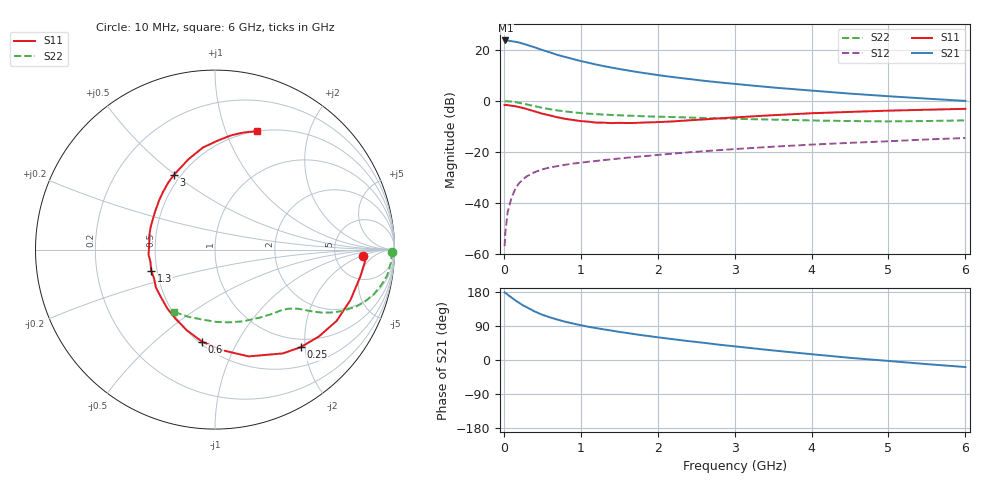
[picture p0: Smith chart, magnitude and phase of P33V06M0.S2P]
! SIEMENS Small Signal Semiconductors
! BFP181
! Si NPN RF Bipolar Junction Transistor in SOT143
! VCE = 3 V  IC = 6 mA
! Common Emitter S-Parameters:  March  1996
# GHz  S  MA  R  50
!  f  S11  S21  S12  S22
! GHz  MAG  ANG  MAG  ANG  MAG  ANG  MAG  ANG
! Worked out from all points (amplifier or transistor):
!   36 points, 10 MHz to 6 GHz, reference 50 ohm
!   highest |S21| = 23.8 dB at 20 MHz (marker M1)
!   |S21| within 3 dB of that: start of sweep to 429.1 MHz
!   unconditionally stable (mu >= 1): 1.539 GHz to end of sweep
!   at 250 MHz: K = 0.25, MSG = 26.6 dB, |S12| = -30.8 dB
!   at 1.4 GHz: K = 0.96, MSG = 18.0 dB, |S12| = -22.9 dB
!   at 6 GHz: K = 1.04, MAG = 6.1 dB, |S12| = -14.6 dB
!   S11 on the Smith chart (normalised r, x): 10 MHz: 10, -2; 250 MHz: 0.84, -1.91; 600 MHz: 0.52, -0.73; 1.3 GHz: 0.46, -0.13; 3 GHz: 0.46, +0.49; 6 GHz: 0.50, +1.29
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0.01  0.8276 -2.3  15.42 178.4  0.0014 84.1  0.9869 -0.8
0.02  0.8391 -4.3  15.43 177.3  0.0026 95.9  0.9863 -1.7
0.05  0.8248 -10.1  15.33 172.3  0.0066 88.4  0.9826 -4.3
0.1  0.8053 -20.4  14.93 164.8  0.0125 79.1  0.9703 -8.5
0.15  0.7857 -30.3  14.51 157.4  0.0189 74.0  0.9455 -12.3
0.2  0.7549 -39.8  14.05 150.6  0.0244 69.7  0.9177 -15.9
0.25  0.7237 -48.7  13.3 144.0  0.0288 64.8  0.8838 -19.1
0.4  0.6239 -72.5  11.31 128.1  0.0398 56.5  0.7893 -25.7
0.5  0.561 -86.2  10.02 119.4  0.0452 51.9  0.7327 -28.6
0.6  0.5184 -97.9  8.998 112.5  0.0495 48.8  0.687 -30.7
0.7  0.476 -109.3  7.991 106.4  0.0524 47.0  0.6506 -32.1
0.8  0.4441 -119.5  7.298 100.9  0.0557 45.0  0.6227 -33.2
0.9  0.4221 -129.0  6.648 96.2  0.0588 44.0  0.5977 -34.1
1.1  0.3912 -147.3  5.626 87.6  0.0639 43.1  0.5623 -35.8
1.3  0.3742 -161.8  4.821 80.8  0.0688 42.2  0.5385 -37.6
1.7  0.3694 171.8  3.768 68.3  0.0791 41.6  0.5078 -41.4
2.2  0.3957 147.3  2.937 54.8  0.0923 39.8  0.4814 -47.6
3  0.4742 119.1  2.162 36.0  0.1132 36.1  0.4453 -59.6
3.5  0.5245 106.4  1.836 25.2  0.1261 33.4  0.4295 -68.5
4.5  0.6088 88.3  1.393 5.7  0.1501 26.6  0.4025 -89.5
5.5  0.6715 76.3  1.109 -10.9  0.175 20.4  0.4031 -112.0
6  0.6995 70.6  1.001 -18.6  0.187 16.7  0.4146 -123.4
